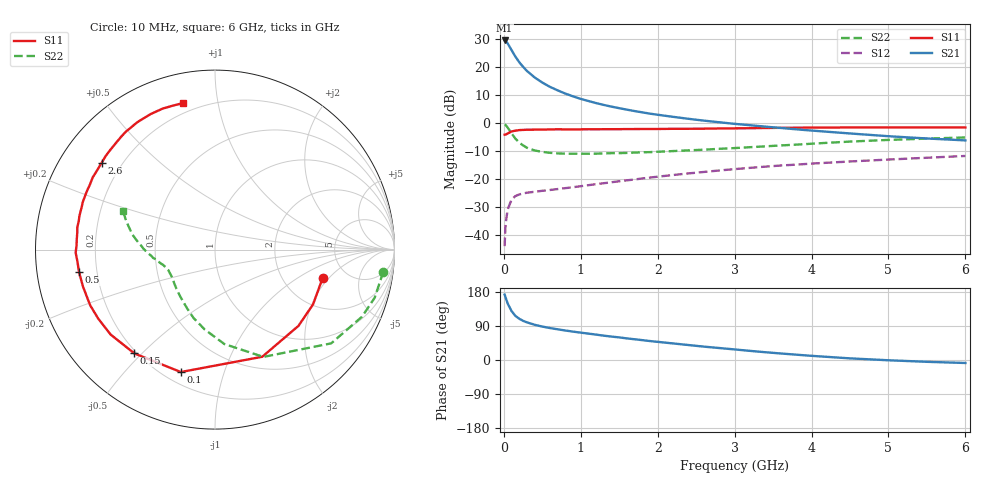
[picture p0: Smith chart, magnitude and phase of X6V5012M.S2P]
! SIEMENS Small Signal Semiconductors
! BFP193W
! Si NPN RF Bipolar Junction Transistor in SOT343
! VCE = 0.5 V  IC = 12 mA
! Common Emitter S-Parameters:  April 1994
# GHz  S  MA  R  50
!  f  S11  S21  S12  S22
! GHz  MAG  ANG  MAG  ANG  MAG  ANG  MAG  ANG
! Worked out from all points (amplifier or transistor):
!   40 points, 10 MHz to 6 GHz, reference 50 ohm
!   highest |S21| = 29.6 dB at 10 MHz (marker M1)
!   |S21| within 3 dB of that: start of sweep to 90.58 MHz
!   unconditionally stable (mu >= 1): 987.5 MHz to end of sweep
!   at 200 MHz: K = 0.28, MSG = 23.7 dB, |S12| = -25.5 dB
!   at 1.5 GHz: K = 1.18, MAG = 10.5 dB, |S12| = -20.8 dB
!   at 6 GHz: K = 1.10, MAG = 0.9 dB, |S12| = -11.8 dB
!   S11 on the Smith chart (normalised r, x): 10 MHz: 3.33, -1.71; 100 MHz: 0.26, -0.72; 150 MHz: 0.19, -0.47; 500 MHz: 0.13, -0.08; 2.6 GHz: 0.13, +0.33; 6 GHz: 0.15, +0.79
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0.01  0.6205 -14.7  30.07 172.6  0.0063 83.9  0.9457 -7.5
0.02  0.6258 -29.2  29.67 166.8  0.0133 77.7  0.9294 -16.7
0.03  0.6299 -42.4  28.88 160.6  0.0186 72.0  0.9007 -24.5
0.05  0.6525 -66.2  26.51 149.1  0.0285 61.4  0.8318 -38.9
0.1  0.7083 -105.6  20.23 129.1  0.0429 45.2  0.6559 -65.7
0.15  0.7325 -127.9  15.49 116.6  0.0495 36.1  0.5289 -84.3
0.2  0.7498 -140.9  12.3 108.9  0.053 31.5  0.4485 -97.4
0.25  0.7558 -149.4  10.17 103.4  0.0552 28.9  0.3994 -107.4
0.3  0.7615 -155.9  8.579 99.3  0.0569 27.8  0.3629 -115.3
0.4  0.764 -164.4  6.563 93.0  0.0591 26.9  0.3248 -126.7
0.5  0.7678 -170.6  5.311 88.2  0.0616 28.0  0.3058 -134.7
0.6  0.7693 -175.0  4.447 84.3  0.0637 29.3  0.2943 -140.7
0.8  0.7717 178.2  3.37 77.8  0.0687 32.2  0.2841 -148.3
1.1  0.7771 170.7  2.483 69.6  0.0776 36.3  0.2835 -155.1
1.3  0.7782 166.2  2.113 64.2  0.0842 38.5  0.287 -157.8
1.6  0.7828 160.3  1.741 57.0  0.0948 40.9  0.2931 -161.0
2.2  0.7911 149.5  1.295 43.7  0.118 42.5  0.3162 -166.8
2.6  0.7954 142.6  1.108 35.3  0.1338 42.2  0.3346 -170.7
3.2  0.8106 133.0  0.917 24.1  0.1584 40.2  0.3709 -176.4
4.5  0.8358 115.5  0.653 4.3  0.206 33.2  0.4676 169.7
5.5  0.8358 106.7  0.531 -4.8  0.2403 27.6  0.5284 160.9
6  0.8355 102.5  0.491 -7.9  0.2585 25.1  0.5539 157.4
